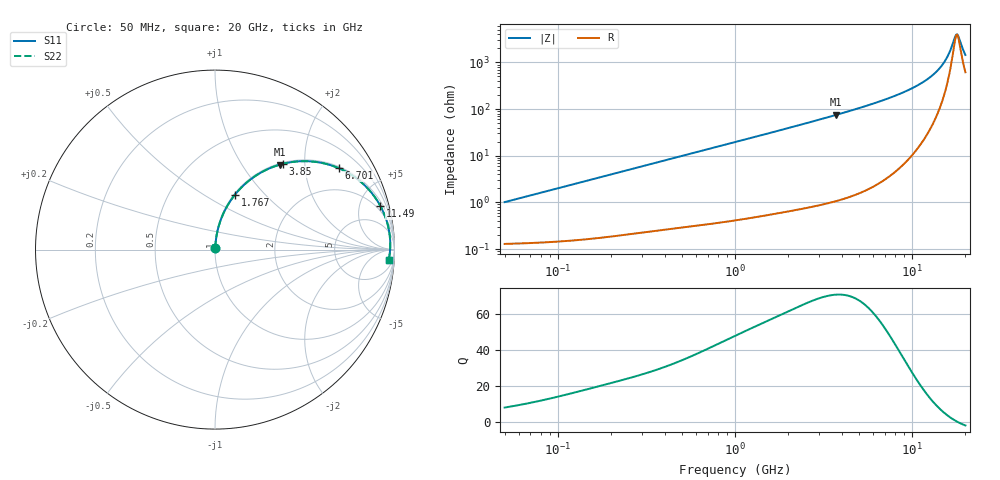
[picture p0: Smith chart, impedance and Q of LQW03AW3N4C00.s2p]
!Murata Part Number: LQW03AW3N4C00
!These Parameters are Measured in Series Mode Connection
!  o--[Z]--o
!Port1  Port2
!  o-------o
!Freq. Start=50[MHz] Stop=20[GHz], 401[Steps]
# Hz S RI R 50
!Freq.(Hz) S11(Real) S11(Imag) S21(Real) S21(Imag) S12(Real) S12(Imag) S22(Real) S22(Imag)
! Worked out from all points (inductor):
!   401 points, 50 MHz to 20 GHz, reference 50 ohm
!   read as one part in series: L = 3.19 nH near 51.52 MHz
!   highest Q = 70.5 at 3.736 GHz (marker M1), where L = 3.2 nH
!   self-resonance near 17.74 GHz
!   S11 on the Smith chart (normalised r, x): 50 MHz: 1.00, +0.02; 1.767 GHz: 1.01, +0.69; 3.85 GHz: 1.02, +1.55; 6.701 GHz: 1.05, +2.99; 11.49 GHz: 1.41, +7.48; 20 GHz: 13, -26
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5e7  0.00138 0.01  0.9986 -0.01  0.9986 -0.01  0.00138 0.01
1.364002e8  0.00231 0.0271  0.9977 -0.0271  0.9977 -0.0271  0.00231 0.0271
3.721004e8  0.00778 0.0724  0.9922 -0.0724  0.9922 -0.0724  0.00778 0.0724
1e9  0.0403 0.1863  0.9597 -0.1863  0.9597 -0.1863  0.0403 0.1863
1.766834e9  0.1105 0.3052  0.8895 -0.3052  0.8895 -0.3052  0.1105 0.3052
2.728004e9  0.2282 0.4123  0.7718 -0.4123  0.7718 -0.4123  0.2282 0.4123
3.736399e9  0.3631 0.4739  0.6369 -0.4739  0.6369 -0.4739  0.3631 0.4739
3.850025e9  0.3781 0.4779  0.6219 -0.4779  0.6219 -0.4779  0.3781 0.4779
5.117541e9  0.534 0.4914  0.466 -0.4914  0.466 -0.4914  0.534 0.4914
6.701223e9  0.6884 0.4541  0.3116 -0.4541  0.3116 -0.4541  0.6884 0.4541
7.442007e9  0.7447 0.4257  0.2553 -0.4257  0.2553 -0.4257  0.7447 0.4257
9.457416e9  0.8559 0.3355  0.1441 -0.3355  0.1441 -0.3355  0.8559 0.3355
1.149051e10  0.9219 0.2424  0.0781 -0.2424  0.0781 -0.2424  0.9219 0.2424
1.334722e10  0.9554 0.1633  0.0446 -0.1633  0.0446 -0.1633  0.9554 0.1633
1.482269e10  0.9696 0.1058  0.0304 -0.1058  0.0304 -0.1058  0.9696 0.1058
1.597544e10  0.975 0.0643  0.025 -0.0643  0.025 -0.0643  0.975 0.0643
1.721783e10  0.9765 0.0228  0.0235 -0.0228  0.0235 -0.0228  0.9765 0.0228
1.774144e10  0.976 0.00624  0.024 -0.00624  0.024 -0.00624  0.976 0.00624
1.800918e10  0.9755 -0.002  0.0245 0.002  0.0245 0.002  0.9755 -0.002
1.828096e10  0.9749 -0.0102  0.0251 0.0102  0.0251 0.0102  0.9749 -0.0102
1.940974e10  0.9708 -0.0428  0.0292 0.0428  0.0292 0.0428  0.9708 -0.0428
2e10  0.9678 -0.0589  0.0322 0.0589  0.0322 0.0589  0.9678 -0.0589
